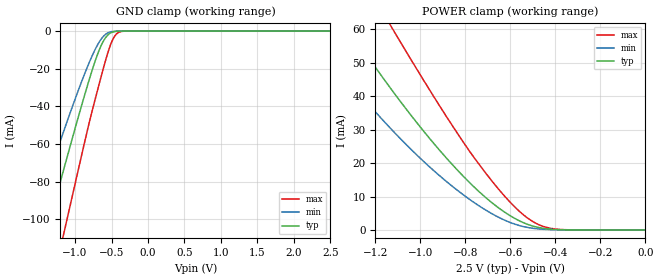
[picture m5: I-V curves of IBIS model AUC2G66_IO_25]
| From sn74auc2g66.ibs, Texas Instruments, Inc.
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[Model]   AUC2G66_IO_25
Model_type  Terminator
| variable   typ   min   max
C_comp   3.43pF   3.07pF   3.66pF
| C_tri-state   3.43pF   3.07pF   3.66pF
[Temperature Range]   40   100   -40
| Ambient temperature   25   85   -40
[Voltage range]   2.5   2.3   2.7
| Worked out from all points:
|   GND clamp passes 1 mA (typ) near -0.51 V on its own axis
|   POWER clamp passes 1 mA (typ) near -0.49 V on its own axis
[GND Clamp]
| AUC2G66_IO_25
|   Voltage   I(typ)   I(min)   I(max)
-2.7V     -295.9mA   -240.2mA   -365.2mA
-1.625V   -141mA     -108.1mA   -187.1mA
-1.58V    -134.5mA   -102.7mA   -179.5mA
-1.37V    -104.2mA   -77.84mA   -144.2mA
-1.155V   -73.53mA   -53.19mA   -107.7mA
-1.12V    -68.58mA   -49.29mA   -101.8mA
-740mV    -17.77mA   -11.02mA   -38.6mA
-640mV    -7.505mA   -4.181mA   -23.83mA
-550mV    -2.079mA   -943.6uA   -11.48mA
-455mV    -253.8uA   -102.1uA   -2.606mA
-340mV    -9.524uA   -4.927uA   -94.63uA
2.5V      757.5pA    256.7nA    851.4pA
[POWER Clamp]
| AUC2G66_IO_25
|   Voltage   I(typ)   I(min)   I(max)
-2.7V     217.7mA    187.7mA    248.3mA
-1.49V    77.66mA    59.08mA    102.8mA
-1.32V    60.26mA    44.66mA    82.76mA
-1.13V    42.11mA    30.16mA    60.84mA
-1.105V   39.85mA    28.4mA     58.01mA
-935mV    25.42mA    17.4mA     39.25mA
-790mV    14.73mA    9.55mA     24.33mA
-645mV    6.229mA    3.535mA    11.58mA
-530mV    1.841mA    833.9uA    3.874mA
-470mV    668.2uA    277.2uA    1.462mA
-390mV    106.5uA    46.38uA    213.7uA
-35.59fV  757.5pA    1.096nA    1.053nA
